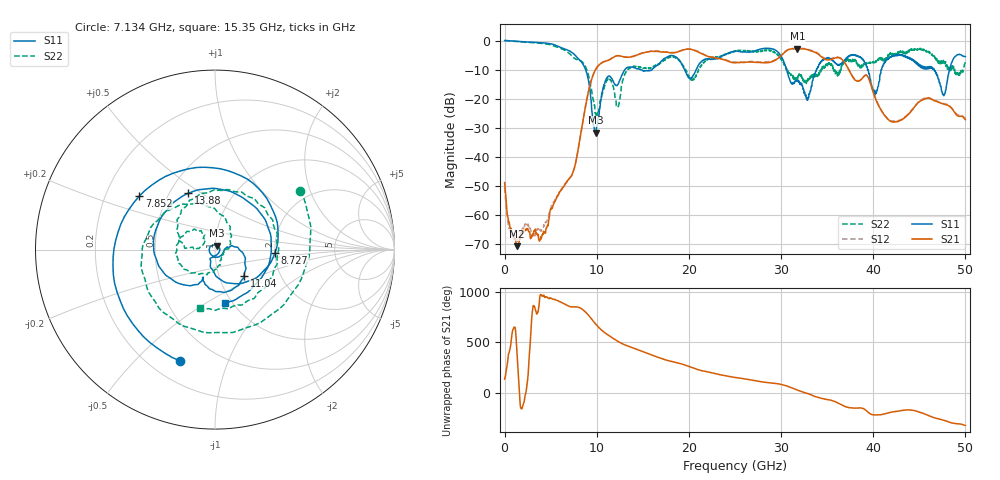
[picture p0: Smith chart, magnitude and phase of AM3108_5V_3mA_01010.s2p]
# Hz S DB R 50.0
!freq dBS11 angS11 dBS21 angS21 dBS12 angS12 dBS22 angS22
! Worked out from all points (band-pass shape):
!   1601 points, 10 MHz to 50 GHz, reference 50 ohm
!   highest |S21| = -2.84 dB at 31.78 GHz (marker M1); lowest = -70.9 dB at 1.322 GHz (marker M2)
!   |S21| within 3 dB of the highest: 11.79 GHz to 22.62 GHz (10.83 GHz wide, 62.9 % of centre); 29.8 GHz to 34.46 GHz (4.663 GHz wide, 14.5 % of centre)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
!   lowest |S11| = -31.8 dB at 9.883 GHz (marker M3), VSWR 1.05, Z = 51.2 + j2.31 ohm
!   |S11| at or under -10 dB: 8.795 GHz to 13.07 GHz (4.277 GHz wide, 39.1 % of centre); 30.61 GHz to 33.84 GHz (3.235 GHz wide, 10 % of centre); 46.63 GHz to 48.28 GHz (1.655 GHz wide, 3.49 % of centre)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
!   |S22| runs from -26.0 to 0.0 dB; largest |S21 - S12| = 0.023
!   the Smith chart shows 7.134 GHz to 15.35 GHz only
!   S11 on the Smith chart (normalised r, x): 7.134 GHz: 0.32, -0.68; 7.852 GHz: 0.35, +0.28; 8.727 GHz: 2.00, -0.07; 11.04 GHz: 1.31, -0.41; 13.88 GHz: 0.62, +0.44; 15.35 GHz: 0.93, -0.60
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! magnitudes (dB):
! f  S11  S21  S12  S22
! 10 MHz  0.0  -49.0  -50.6  0.0
! 1.322 GHz  -0.3  -70.9  -68.7  -0.4
! 3.947 GHz  -0.8  -67.8  -65.7  -1.0
! 7.134 GHz  -3.7  -47.1  -47.2  -4.8
! 7.852 GHz  -5.7  -39.9  -40.1  -6.6
! 8.352 GHz  -7.4  -30.7  -30.7  -7.1
! 8.727 GHz  -9.5  -23.8  -23.6  -8.6
! 9.883 GHz  -31.8  -10.0  -9.9  -24.8
! 11.04 GHz  -13.2  -7.0  -7.0  -14.3
! 12.29 GHz  -15.2  -5.2  -5.2  -22.9
! 13.88 GHz  -9.2  -5.6  -5.4  -8.9
! 15.35 GHz  -10.4  -4.0  -4.0  -9.5
! 16.69 GHz  -8.2  -3.8  -3.6  -8.3
! 20.41 GHz  -12.2  -3.2  -3.2  -13.7
! 25 GHz  -3.7  -7.7  -7.4  -3.8
! 31.78 GHz  -14.1  -2.8  -2.6  -13.4
! 33.35 GHz  -15.5  -3.7  -3.4  -12.7
! 37.88 GHz  -4.8  -13.1  -12.9  -6.4
! 40.22 GHz  -18.7  -19.9  -19.6  -7.6
! 41.69 GHz  -6.1  -27.4  -27.3  -5.4
! 47.66 GHz  -19.0  -21.9  -21.8  -7.7
! 50 GHz  -5.5  -27.3  -26.9  -6.9
